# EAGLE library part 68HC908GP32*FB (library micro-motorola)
MC68HC908GP32 MC68HC08GP32 Source: www.motorola.com .. MC68HC908GP32.pdf
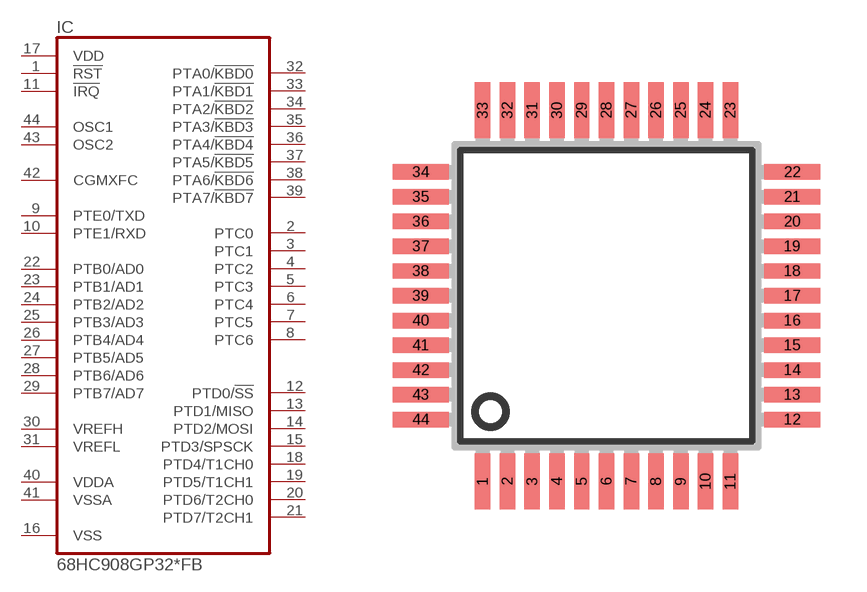
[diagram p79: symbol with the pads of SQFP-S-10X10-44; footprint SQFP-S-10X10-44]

Designator prefix IC

## 68HC908GP32CFB (MF: MOTOROLA; MPN: MC68HC908GP32CFB; OC_FARNELL: unknown; OC_NEWARK: 02C6745), 68HC908GP32MFB (OC_FARNELL: unknown; OC_NEWARK: unknown), 68HC908GP32VFB (OC_FARNELL: unknown; OC_NEWARK: unknown)  [SQFP-S-10X10-44]
1  !RST  in
2  PTC0
3  PTC1
4  PTC2
5  PTC3
6  PTC4
7  PTC5
8  PTC6
9  PTE0/TXD
10  PTE1/RXD
11  !IRQ  in
12  PTD0/!SS
13  PTD1/MISO
14  PTD2/MOSI
15  PTD3/SPSCK
16  VSS  pwr
17  VDD  pwr
18  PTD4/T1CH0
19  PTD5/T1CH1
20  PTD6/T2CH0
21  PTD7/T2CH1
22  PTB0/AD0
23  PTB1/AD1
24  PTB2/AD2
25  PTB3/AD3
26  PTB4/AD4
27  PTB5/AD5
28  PTB6/AD6
29  PTB7/AD7
30  VREFH  in
31  VREFL  in
32  PTA0/!KBD0
33  PTA1/!KBD1
34  PTA2/!KBD2
35  PTA3/!KBD3
36  PTA4/!KBD4
37  PTA5/!KBD5
38  PTA6/!KBD6
39  PTA7/!KBD7
40  VDDA  pwr
41  VSSA  pwr
42  CGMXFC  in
43  OSC2  in
44  OSC1  in

## Footprint SQFP-S-10X10-44 (pad centres in mm)
QFP44 shrink quad flat pack, square
smd 0.5 x 1.8: 1 -4,-6; 2 -3.2,-6; 3 -2.4,-6; 4 -1.6,-6; 5 -0.8,-6; 6 0,-6; 7 0.8,-6; 8 1.6,-6; 9 2.4,-6; 10 3.2,-6; 11 4,-6; 23 4,6; 24 3.2,6; 25 2.4,6; 26 1.6,6; 27 0.8,6; 28 0,6; 29 -0.8,6; 30 -1.6,6; 31 -2.4,6; 32 -3.2,6; 33 -4,6
smd 1.8 x 0.5: 12 6,-4; 13 6,-3.2; 14 6,-2.4; 15 6,-1.6; 16 6,-0.8; 17 6,0; 18 6,0.8; 19 6,1.6; 20 6,2.4; 21 6,3.2; 22 6,4; 34 -6,4; 35 -6,3.2; 36 -6,2.4; 37 -6,1.6; 38 -6,0.8; 39 -6,0; 40 -6,-0.8; 41 -6,-1.6; 42 -6,-2.4; 43 -6,-3.2; 44 -6,-4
